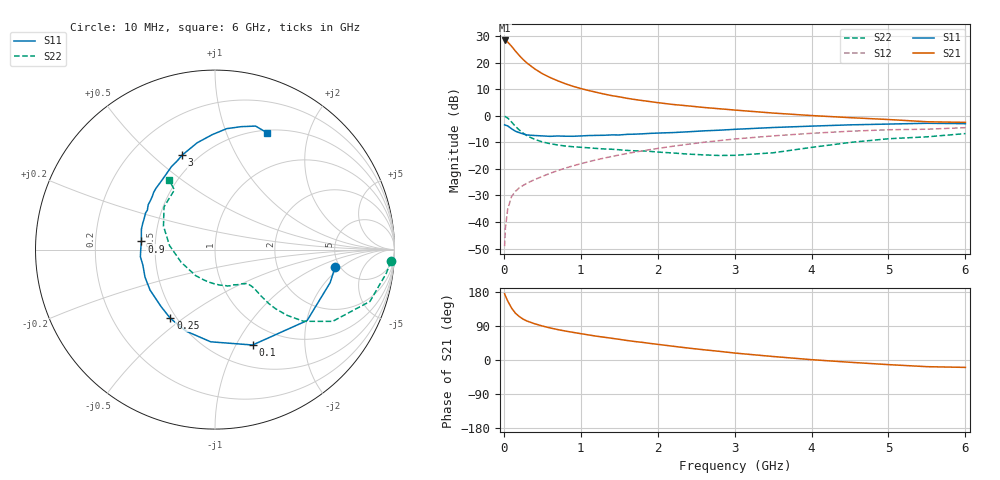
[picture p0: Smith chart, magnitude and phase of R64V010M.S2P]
! SIEMENS Small Signal Semiconductors
! BFR193
! Si NPN RF Bipolar Junction Transistor in SOT23
! VCE = 4 V  IC = 10 mA
! Common Emitter S-Parameters:  May  1996
# GHz  S  MA  R  50
!  f  S11  S21  S12  S22
! GHz  MAG  ANG  MAG  ANG  MAG  ANG  MAG  ANG
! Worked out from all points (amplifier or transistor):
!   36 points, 10 MHz to 6 GHz, reference 50 ohm
!   highest |S21| = 28.4 dB at 10 MHz (marker M1)
!   |S21| within 3 dB of that: start of sweep to 123 MHz
!   unconditionally stable (mu >= 1): 742.4 MHz to 1.958 GHz
!   at 250 MHz: K = 0.64, MSG = 23.7 dB, |S12| = -26.2 dB
!   at 1.4 GHz: K = 1.04, MAG = 10.3 dB, |S12| = -15.3 dB
!   at 6 GHz: K = 0.95, MSG = 1.0 dB, |S12| = -4.5 dB
!   lowest NFmin = 1.30 dB at 450 MHz
!   S11 on the Smith chart (normalised r, x): 10 MHz: 4.61, -1.60; 100 MHz: 0.74, -1.17; 250 MHz: 0.46, -0.45; 900 MHz: 0.42, +0.05; 3 GHz: 0.41, +0.63; 6 GHz: 0.53, +1.40
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0.01  0.6768 -8.0  26.37 174.9  0.0035 88.7  0.9821 -3.8
0.02  0.6675 -16.0  26.29 169.6  0.0076 81.4  0.9638 -7.8
0.05  0.6478 -37.6  24.58 155.8  0.0174 73.2  0.9103 -18.5
0.1  0.5713 -68.5  20.54 137.2  0.03 63.5  0.7676 -31.4
0.15  0.5142 -92.7  16.69 123.6  0.0377 58.1  0.6347 -39.0
0.2  0.4821 -109.6  13.76 114.8  0.044 56.0  0.5428 -42.4
0.25  0.4567 -123.0  11.54 107.9  0.0488 55.3  0.4727 -44.3
0.3  0.4369 -133.6  9.93 102.9  0.0538 56.4  0.4233 -45.1
0.4  0.4264 -148.1  7.708 95.7  0.0629 57.7  0.3609 -45.2
0.5  0.4191 -158.5  6.242 89.7  0.0723 59.4  0.3229 -44.8
0.6  0.411 -168.1  5.288 84.7  0.0825 60.9  0.299 -44.8
0.7  0.4176 -174.6  4.584 80.3  0.093 62.0  0.2827 -45.2
0.9  0.4123 173.7  3.603 72.9  0.1144 62.8  0.2615 -46.5
1.1  0.4255 164.5  3.009 66.2  0.1366 62.9  0.25 -49.7
1.3  0.4306 156.5  2.581 60.2  0.1596 62.1  0.2382 -53.4
1.6  0.4482 146.1  2.145 51.5  0.1951 60.4  0.2234 -61.4
2.2  0.4843 128.4  1.638 36.3  0.268 54.6  0.1996 -82.2
3  0.5575 109.1  1.287 18.4  0.3661 43.9  0.1805 -126.8
3.5  0.6032 99.5  1.129 9.2  0.4194 36.4  0.2014 -159.5
4.5  0.6769 84.5  0.925 -6.0  0.5136 21.4  0.3154 155.5
5.5  0.7245 71.8  0.774 -17.6  0.5604 5.9  0.4022 124.2
6  0.7127 66.2  0.754 -19.5  0.5989 1.4  0.4634 123.4
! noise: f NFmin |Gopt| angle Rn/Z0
0.45  1.3  0.22  143  0.11
0.9  1.3  0.34  160  0.11
1.8  2.05  0.54  -153  0.14
